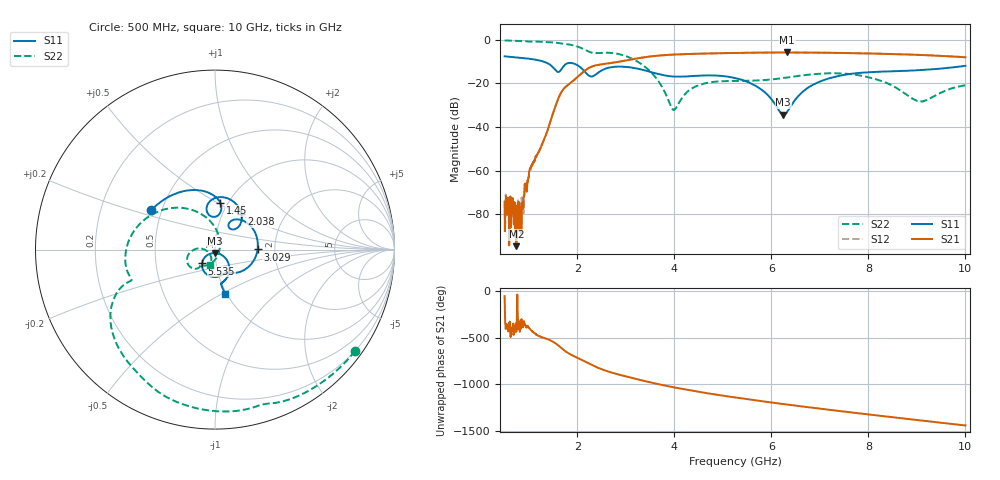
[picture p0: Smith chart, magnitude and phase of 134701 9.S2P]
!  2-Port S-parameters saved by WinCal
! VAR MeasName=S-Parameters (CALIBRATED_DATA) read from VNA (N5242A)
! VAR MeasDate=2013-7-3 16:27:44
! VAR NAME=134701 9
! VAR FILENAME=134701 9.S2P
! VAR DATE=2013-7-3 16:27:45
! VAR PHYS_PORTS=1,2
# Hz S MA R 50
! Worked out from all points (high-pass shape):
!   1601 points, 500 MHz to 10 GHz, reference 50 ohm
!   highest |S21| = -5.82 dB at 6.325 GHz (marker M1); lowest = -94.5 dB at 743.4 MHz (marker M2)
!   |S21| within 3 dB of the highest: 3.162 GHz to end of sweep
!   lowest |S11| = -34.3 dB at 6.242 GHz (marker M3), VSWR 1.04, Z = 49.8 - j1.92 ohm
!   |S11| at or under -10 dB: 1.3 GHz to end of sweep
!   |S22| runs from -32.2 to -0.3 dB; largest |S21 - S12| = 0.0024
!   S11 on the Smith chart (normalised r, x): 500 MHz: 0.44, +0.23; 1.45 GHz: 0.92, +0.52; 2.038 GHz: 1.23, +0.52; 3.029 GHz: 1.62, +0.00; 5.535 GHz: 0.86, -0.13; 10 GHz: 0.98, -0.52
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5e8  0.4178 148.3  0.000191 -53.7  0.0002086 -2.0  0.9635 -35.9
7.434375e8  0.3956 133.9  1.879e-05 -74.4  7.064e-05 -47.9  0.9477 -53.2
8.44375e8  0.3856 127.7  3.663e-05 53.0  4.928e-05 59.4  0.9379 -60.4
1.052188e9  0.3616 114.1  0.001319 -64.5  0.001218 -64.7  0.9026 -74.0
1.45e9  0.2612 83.3  0.01422 -169.1  0.0142 -169.4  0.8774 -103.1
1.681562e9  0.2209 102.1  0.06621 104.5  0.06599 104.2  0.8169 -120.7
2.037812e9  0.2463 53.2  0.1524 -5.1  0.152 -5.1  0.6765 -149.3
2.085312e9  0.2228 48.0  0.1699 -17.3  0.1694 -17.3  0.6428 -152.7
2.269375e9  0.1447 52.0  0.2351 -65.5  0.2348 -65.4  0.5177 -159.5
2.4475e9  0.1823 60.7  0.2684 -107.6  0.268 -107.5  0.4961 -161.7
3.029375e9  0.2373 0.2  0.3398 160.5  0.3396 160.6  0.4103 152.9
3.670625e9  0.1643 -52.8  0.4339 81.4  0.4336 81.4  0.1129 86.7
3.99125e9  0.1438 -63.8  0.4577 46.9  0.4581 46.9  0.02498 -13.9
4.436562e9  0.149 -78.3  0.4769 4.8  0.4774 4.8  0.08485 -108.5
5.25e9  0.133 -119.3  0.4985 -61.2  0.4986 -61.2  0.1145 -132.8
5.535e9  0.1055 -133.2  0.5044 -82.2  0.504 -82.3  0.1156 -133.7
6.241562e9  0.01936 -95.6  0.5107 -131.7  0.5109 -131.7  0.1329 -131.6
6.324688e9  0.02243 -64.0  0.5116 -137.3  0.5106 -137.3  0.1367 -131.9
6.835312e9  0.09012 -41.8  0.5078 -171.0  0.5077 -170.9  0.1612 -139.0
8.420625e9  0.1887 -78.1  0.4741 91.3  0.4735 91.4  0.09772 176.4
9.067812e9  0.202 -79.8  0.4482 52.9  0.4488 52.8  0.039 -147.1
1e10  0.2531 -77.6  0.3971 -1.8  0.3981 -1.7  0.09037 -109.2
